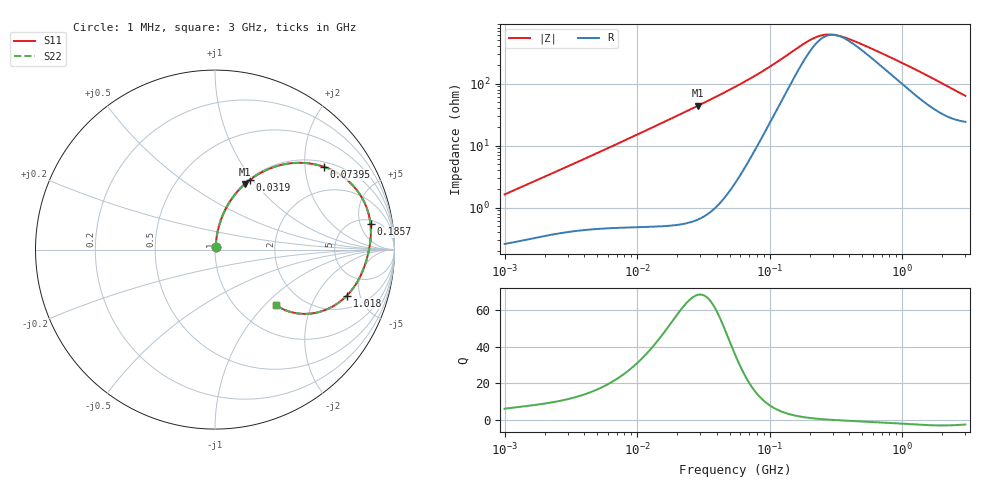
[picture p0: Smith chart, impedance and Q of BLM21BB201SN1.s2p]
! BLM21BB201SN1
# Hz S RI R 50
!Freq.(Hz) S11(Real) S11(Imag) S21(Real) S21(Imag) S12(Real) S12(Imag) S22(Real) S22(Imag)
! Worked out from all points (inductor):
!   401 points, 1 MHz to 3 GHz, reference 50 ohm
!   read as one part in series: L = 254 nH near 1.041 MHz
!   highest Q = 68.3 at 28.87 MHz (marker M1), where L = 243 nH
!   self-resonance near 313 MHz
!   S11 on the Smith chart (normalised r, x): 1 MHz: 1.01, +0.03; 31.9 MHz: 1.01, +0.98; 73.95 MHz: 1.14, +2.52; 185.7 MHz: 6.11, +7.48; 1.018 GHz: 2.90, -3.76; 3 GHz: 1.48, -1.17
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1000000  0.00285 0.016  0.9972 -0.016  0.9972 -0.016  0.00285 0.016
3823119  0.00763 0.0576  0.9924 -0.0576  0.9924 -0.0576  0.00763 0.0576
7858845  0.0183 0.1154  0.9817 -0.1154  0.9817 -0.1154  0.0183 0.1154
1.461624e7  0.0504 0.2076  0.9496 -0.2076  0.9496 -0.2076  0.0504 0.2076
2.095589e7  0.0951 0.285  0.9049 -0.285  0.9049 -0.285  0.0951 0.285
2.886629e7  0.1662 0.365  0.8338 -0.365  0.8338 -0.365  0.1662 0.365
3.190472e7  0.1967 0.3902  0.8033 -0.3902  0.8033 -0.3902  0.1967 0.3902
4.138676e7  0.2977 0.4486  0.7023 -0.4486  0.7023 -0.4486  0.2977 0.4486
5.477226e7  0.4394 0.4826  0.5606 -0.4826  0.5606 -0.4826  0.4394 0.4826
7.395247e7  0.6075 0.4609  0.3925 -0.4609  0.3925 -0.4609  0.6075 0.4609
1.148668e8  0.7972 0.3221  0.2028 -0.3221  0.2028 -0.3221  0.7972 0.3221
1.857042e8  0.8665 0.1405  0.1335 -0.1405  0.1335 -0.1405  0.8665 0.1405
2.094008e8  0.8686 0.1029  0.1314 -0.1029  0.1314 -0.1029  0.8686 0.1029
2.609752e8  0.8651 0.0429  0.1349 -0.0429  0.1349 -0.0429  0.8651 0.0429
3.252521e8  0.8566 -0.00855  0.1434 0.00855  0.1434 0.00855  0.8566 -0.00855
4.304467e8  0.8412 -0.0678  0.1588 0.0678  0.1588 0.0678  0.8412 -0.0678
8.005644e8  0.7794 -0.2012  0.2206 0.2012  0.2206 0.2012  0.7794 -0.2012
1.017911e9  0.7345 -0.2563  0.2655 0.2563  0.2655 0.2563  0.7345 -0.2563
1.374365e9  0.651 -0.3194  0.349 0.3194  0.349 0.3194  0.651 -0.3194
1.855641e9  0.5354 -0.3562  0.4646 0.3562  0.4646 0.3562  0.5354 -0.3562
2.312676e9  0.4408 -0.3523  0.5592 0.3523  0.5592 0.3523  0.4408 -0.3523
3e9  0.3414 -0.3108  0.6586 0.3108  0.6586 0.3108  0.3414 -0.3108
